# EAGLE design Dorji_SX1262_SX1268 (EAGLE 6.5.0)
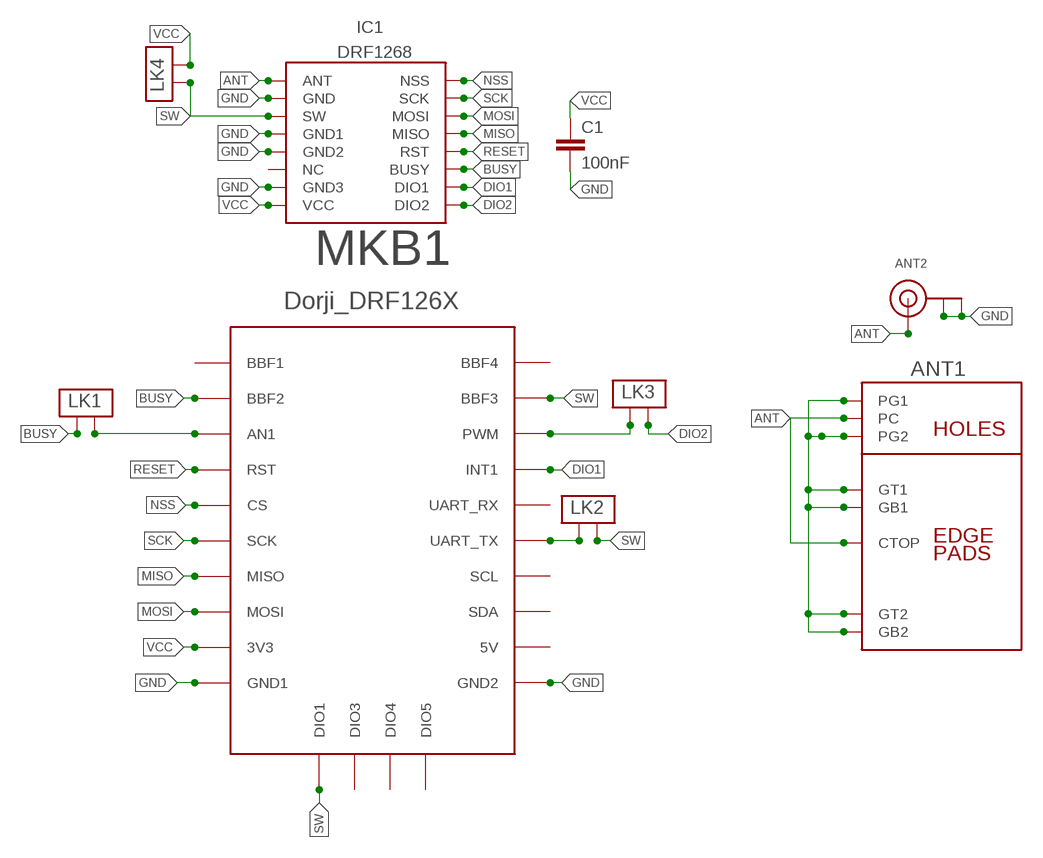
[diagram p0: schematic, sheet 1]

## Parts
ANT1  CUSTOMSMA  [CUSTOMSMA]
ANT2  ANTENNA_U.FL  [U.FL]
C1  100nF  C-EUC1206  [C1206]
IC1  DRF1268  [DRF1268]
LK1  PCB_LINK  [PCB_LINK]
LK2  PCB_LINK  [PCB_LINK]
LK3  PCB_LINK  [PCB_LINK]
LK4  PCB_LINK  [PCB_LINK]
MKB1  BOARD_BBFRIENDLY  [BOARD_BBFRIENDLY]

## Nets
ANT: ANT1.CTOP ANT1.PC ANT2.3(SIGNAL) IC1.1(ANT)
BUSY: IC1.11(BUSY) LK1.P$2 MKB1.BBF2
DIO1: IC1.10(DIO1) MKB1.INT(INT1)
DIO2: IC1.9(DIO2) LK3.P$1
GND [VDD]: ANT1.G1 ANT1.G2 ANT1.GB1 ANT1.GB2 ANT1.GT1 ANT1.GT2 ANT2.1(GND) ANT2.2(GND) C1.2 IC1.2(GND) IC1.4(GND1) IC1.5(GND2) IC1.7(GND3) MKB1.GND1 MKB1.GND2
MISO: IC1.13(MISO) MKB1.MISO
MOSI: IC1.14(MOSI) MKB1.MOSI
N$1: LK2.P$2 MKB1.TX(UART_TX)
N$2: LK3.P$2 MKB1.PWM
N$3: LK1.P$1 MKB1.AN1
NSS: IC1.16(NSS) MKB1.CS
RESET: IC1.12(RST) MKB1.RST
SCK: IC1.15(SCK) MKB1.SCK
SW: IC1.3(SW) LK2.P$1 LK4.P$2 MKB1.BBF3 MKB1.DIO1
VCC [VDD]: C1.1 IC1.8(VCC) LK4.P$1 MKB1.3V3
Unconnected: IC1.6(NC) MKB1.5V MKB1.BBF1 MKB1.BBF4 MKB1.DIO3 MKB1.DIO4 MKB1.DIO5 MKB1.RX(UART_RX) MKB1.SCL MKB1.SDA

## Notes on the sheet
- Dorji_DRF126X

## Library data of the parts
ANT1 = con-coax:CUSTOMSMA
ANT2 = adafruit:ANTENNA_U.FL: U.FL Antenna Connector
C1 = resistor:C-EU: CAPACITOR, European symbol
IC1 = LMA2:DRF1268
LK1-LK4 = LMA2:PCB_LINK
MKB1 = My_Mikrobus:BOARD_BBFRIENDLY

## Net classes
0 default: width 0.203 mm
1 POWER: width 0.635 mm
2 VDD: width 0.635 mm

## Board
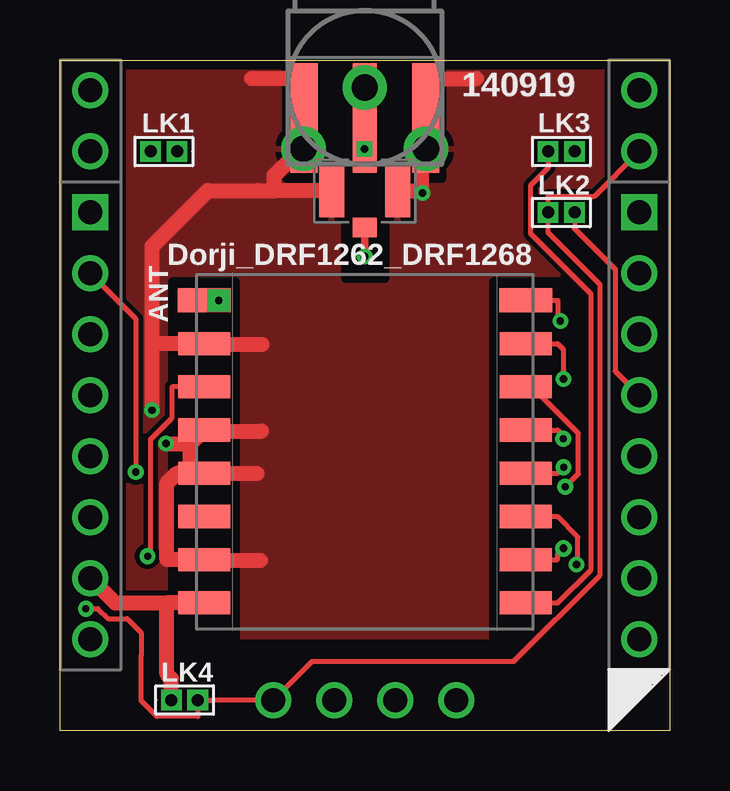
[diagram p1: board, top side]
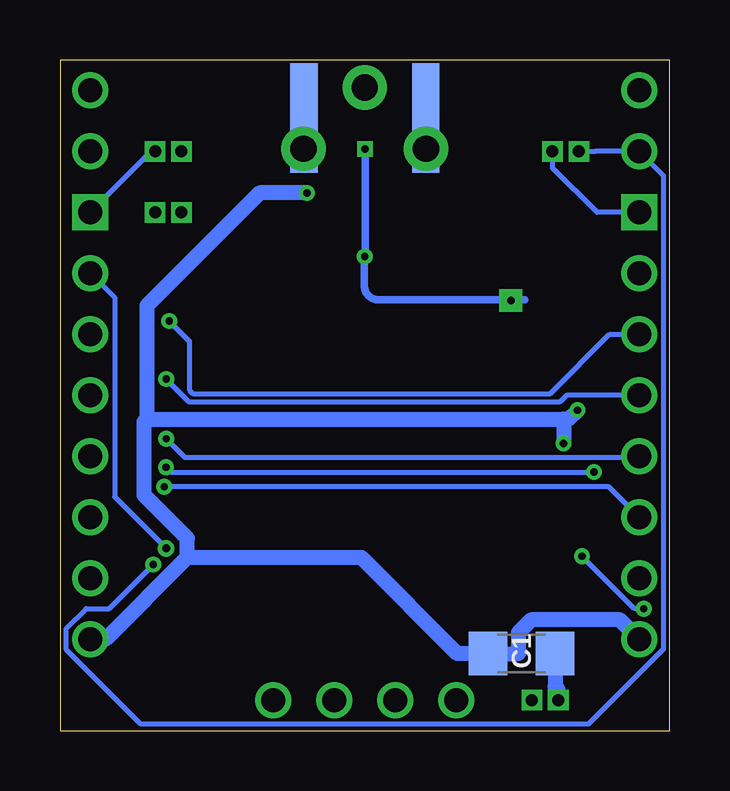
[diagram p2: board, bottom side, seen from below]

Size 25.4 x 27.94 mm. Coordinates in mm from the lower left corner, seen from the top.
Outline: 0,27.93 25.4,27.94 25.4,0 0,0 0,27.93
Copper layers (1*16): Top 0.0356mm / dielectric 1.5011mm / Bottom 0.0356mm
Design rules "LaenPCBOrder *": minimum track width 6mil, minimum drill 13mil, track to track 6mil, track to pad 6mil, pad to pad 6mil, via to via 6mil, smd to smd 6mil, copper to edge 15mil, drill to drill 6mil, minimum pad ring 7mil, minimum via ring 7mil, stop-mask expansion 4mil, vias tented up to drill 0mil, thermal gap 10mil
tRestrict: area 9.4,23 to 15.9,27.9; area 11.8,21.4 to 13.6,23.6; area 11.9,18.8 to 13.5,21.4; area 0,-0.6 to 0.4,27.9; area 25,-0.4 to 25.4,28.1; area 0,2.6 to 2.5,27.9; area 22.9,2.5 to 25.4,27.9; area 7.9,-0.1 to 17.7,2.5; area 4.7,4.5 to 7.3,18.7; area 18.1,4.5 to 20.7,18.7; area 4.7,1.1 to 7.3,4.5; area 18.1,3.1 to 19.9,4.5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
bRestrict: area 5.7,14.3 to 19.8,19; area 9.5,23 to 15.9,27.9; area 10.8,18.9 to 14.6,27.9

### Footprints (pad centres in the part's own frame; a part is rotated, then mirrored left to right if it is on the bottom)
CUSTOMSMA = smd 4.572 x 1.016: CTOP -1.27,0 | drill 1.1 pad 1.85: G1 -2.55,2.55; G2 -2.55,-2.55; PC 0,0 | smd 4.572 x 1.143 bottom: GB1 -1.27,2.54; GB2 -1.27,-2.54 | smd 4.572 x 1.143: GT1 -1.27,2.54; GT2 -1.27,-2.54
U.FL = smd 2.2 x 1.05: 1 0,1.375; 2 0,-1.375 | smd 0.8 x 1: 3 1.525,0
C1206 = smd 1.6 x 1.8: 1 -1.4,0; 2 1.4,0
DRF1268 = smd 2.2 x 1: 1 0.3,12.6; 16 13.7,12.6 | smd 2.159 x 0.965: 2 0.3,10.8; 3 0.3,9; 4 0.3,7.2; 5 0.3,5.4; 6 0.3,3.6; 7 0.3,1.8; 8 0.3,0; 9 13.7,0; 10 13.7,1.8; 11 13.7,3.6; 12 13.7,5.4; 13 13.7,7.2; 14 13.7,9; 15 13.7,10.8
PCB_LINK = drill 0.5 pad 0.813 square: P$1 -0.55,0; P$2 0.55,0
BOARD_BBFRIENDLY = drill 1: 3V3 -11.43,5.08; 5V 11.43,5.08; BBF1 -11.43,25.4; BBF2 -11.43,22.86; BBF3 11.43,22.86; BBF4 11.43,25.4; CS -11.43,15.24; DIO1 -3.81,0; DIO3 -1.27,0; DIO4 1.27,0; DIO5 3.81,0; GND1 -11.43,2.54; GND2 11.43,2.54; INT 11.43,17.78; MISO -11.43,10.16; MOSI -11.43,7.62; RST -11.43,17.78; RX 11.43,15.24; SCK -11.43,12.7; SCL 11.43,10.16; SDA 11.43,7.62; TX 11.43,12.7 | drill 1 square: AN1 -11.43,20.32; PWM 11.43,20.32

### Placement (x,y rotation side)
ANT1  12.7,26.79 90 top
ANT2  12.7,22.49 270 top
C1  6.17,3.21 180 bottom
IC1  5.71,5.32 0 top
LK1  4.33,24.13 180 top
LK2  20.89,21.59 0 top
LK3  20.89,24.13 0 top
LK4  5.19,1.27 0 top
MKB1  12.7,1.27 0 top

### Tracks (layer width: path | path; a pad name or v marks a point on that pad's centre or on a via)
ANT  (via drill 0.3 pad 0.66, 0.3 pad 0.96)
  Top 0.203: ANT1.PC
  Top 0.305: ANT1.CTOP ANT1.PC v12.69,24.23 | v12.7,19.75 ANT2.3 | IC1.1 v6.61,17.92
  Bottom 0.305: v12.69,24.23 v12.69,19.76 v12.7,19.75 12.72,19.73 12.72,18.54 12.72,18.5 12.72,18.47 12.71,18.43 12.7,18.4 12.69,18.36 12.68,18.33 12.67,18.3 12.65,18.27 12.63,18.23 12.62,18.2 12.59,18.18 12.57,18.15 12.55,18.12 12.52,18.1 12.49,18.08 12.46,18.05 12.44,18.04 12.4,18.02 12.37,18 12.34,17.99 12.31,17.98 12.27,17.97 12.24,17.96 12.2,17.95 12.17,17.95 12.13,17.95 6.07,17.95 6.03,17.95 v6.61,17.92
BUSY  (via drill 0.3 pad 0.66)
  Top 0.203: IC1.11 20.74,8.92 21.58,8.07 21.58,6.98 v21.52,6.92
  Bottom 0.203: v21.52,6.92 23.36,5.08 24.31,5.08 25.14,4.26 25.14,3.37 22.03,0.26 3.38,0.26 0.26,3.38 0.26,23.12 MKB1.BBF2 3.1,24.13 LK1.P$2
DIO1  (via drill 0.33 pad 0.69)
  Top 0.203: IC1.10 20.74,7.12 20.74,7.35 v20.98,7.59
  Bottom 0.203: MKB1.INT 23.13,18.05 23.13,9.74 v20.98,7.59
DIO2
  Top 0.203: IC1.9 20.74,5.32 22.13,6.71 22.13,18.19 19.62,20.7 19.62,22.73 20.34,23.45 LK3.P$1
GND  (via drill 0.3 pad 0.66)
  Top 0.635: v15.11,22.4 15.02,22.49 | 15.02,22.49 15.02,22.62 15.07,22.68 15.07,24.06 ANT1.G2 ANT1.GB2 | ANT2.1 15.02,22.49 | v3.83,13.35 3.83,15.31 3.83,16.2 | 8.93,22.49 8.29,22.49 8.28,22.5 6.15,22.5 3.83,20.18 3.83,16.2 | v4.42,11.96 5.43,11.96 5.43,11.95 | 5.43,11.95 IC1.4 | 5.43,10.72 5.43,11.95 | 5.43,10.72 4.86,10.72 4.46,10.31 4.46,7.12 IC1.7 | IC1.5 5.43,10.72 | 8.93,22.49 8.93,23.12 10.05,24.24 ANT1.G1 ANT1.GB1 | ANT2.2 8.93,22.49 | IC1.2 3.92,16.12 3.83,16.2 | 6.79,16.09 8.42,16.09 | 6.58,10.72 8.21,10.72 | 6.72,7.09 8.35,7.09 | 7.97,27.17 9.6,27.17 | 15.72,27.16 17.35,27.16 | 6.77,12.48 8.4,12.48 6.77,12.48
  Bottom 0.635: 21.78,12.97 4.42,12.97 | 20.09,7.22 20.09,8.01 21.89,9.81 21.89,12.86 21.78,12.97 | v15.11,22.4 17.08,22.4 21.78,17.7 21.78,12.97 | 4.42,12.97 4.22,12.97 v3.83,13.35 | 4.42,12.97 v4.42,11.96 | 20.09,7.22 23.5,3.81 MKB1.GND2 | 20.09,7.22 12.85,7.22 8.84,3.21 C1.2 6.3,3.21 6.3,4.08 5.77,4.61 2.07,4.61 MKB1.GND1 | ANT1.GB1 ANT1.G1 | ANT1.G2 ANT1.GB2
  pour Top (isolate 0.2): 0,0 0,27.94 25.4,27.94 25.4,0
MISO  (via drill 0.3 pad 0.66)
  Top 0.203: v20.97,12.16 20.97,12.29 20.74,12.52 IC1.13
  Bottom 0.203: MKB1.MISO 1.32,11.38 20.18,11.38 v20.97,12.16
MOSI  (via drill 0.3 pad 0.66)
  Top 0.203: v21.05,10.15 21.59,10.69 21.59,12.38 19.66,14.32 IC1.14
  Bottom 0.203: MKB1.MOSI 2.53,10.15 v21.05,10.15
N$1
  Top 0.203: LK2.P$2 21.44,20.91 23.13,19.22 23.13,14.97 MKB1.TX
N$2
  Bottom 0.203: LK3.P$2 21.59,24.13 MKB1.PWM
N$3
  Bottom 0.203: LK1.P$1 4.88,23.45 3.02,21.59 MKB1.AN1
NSS  (via drill 0.3 pad 0.66)
  Top 0.203: v20.85,17.07 20.76,17.16 20.76,17.92 IC1.16
  Bottom 0.203: v20.85,17.07 20.01,16.23 20.01,14.19 19.86,14.04 4.98,14.04 2.51,16.51 MKB1.CS
RESET  (via drill 0.3 pad 0.66)
  Top 0.203: MKB1.RST 3.15,17.17 v3.15,10.77 | v20.98,10.97 20.74,10.72 IC1.12
  Bottom 0.203: v20.98,10.97 20.79,10.77 v3.15,10.77
SCK  (via drill 0.3 pad 0.66)
  Top 0.203: v20.98,14.64 20.98,15.88 20.74,16.12 IC1.15
  Bottom 0.203: MKB1.SCK 4.29,13.97 4.58,13.68 20.01,13.68 v20.98,14.64
SW  (via drill 0.3 pad 0.66)
  Top 0.203: v3.65,7.26 3.78,7.39 3.78,12.14 4.67,13.04 4.67,14.32 IC1.3 | MKB1.BBF3 22.27,22.27 20.34,22.27 LK2.P$1 20.34,20.75 22.51,18.58 22.51,6.48 18.91,2.88 10.5,2.88 MKB1.DIO1 6.42,1.27 LK4.P$2 5.74,0.59 4.04,0.59 3.38,1.25 3.38,3.12 3.38,3.13 3.38,4.08 2.8,4.66 2,4.66 1.58,5.08 1.42,5.08 v1.08,5.08 | v1.08,5.08
  Bottom 0.203: v1.08,5.08 1.47,5.08 v3.65,7.26
VCC
  Top 0.635: LK4.P$1 4.64,2.17 4.46,2.35 4.46,5.32 | MKB1.3V3 2.3,5.32 4.46,5.32 | IC1.8 4.46,5.32
  Bottom 0.635: C1.1 4.77,1.84 4.64,1.71 LK4.P$1

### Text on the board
tPlace: 140919 | LK1 | LK3 | LK2 | Dorji_DRF1262_DRF1268 | ANT | LK4
bPlace: C1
